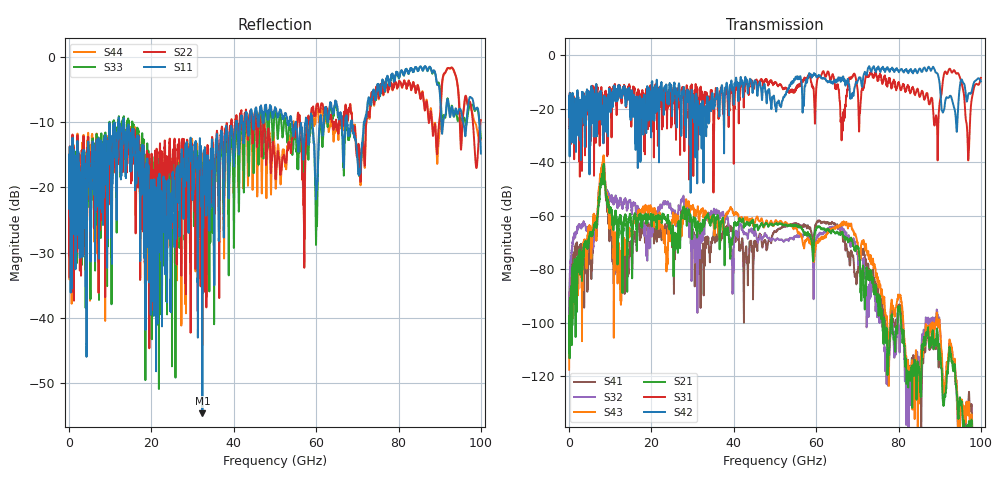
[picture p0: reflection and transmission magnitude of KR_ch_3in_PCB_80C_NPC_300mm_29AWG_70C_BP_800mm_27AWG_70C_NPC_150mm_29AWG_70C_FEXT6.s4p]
# Hz S RI R 45
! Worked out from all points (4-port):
!   4000 points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, 25 MHz to 100 GHz, reference 45 ohm
!   strongest paths, dB at 25 MHz, 25.02 GHz, 50.02 GHz, 75.03 GHz, 100 GHz:
!     S42: -20.7, -20.7, -18.8, -4.2, -9.7
!     S31: -20.7, -20.9, -10.3, -8.7, -8.4
!     S21: -108.7, -69.4, -63.1, -91.8, -168.8
!     S43: -117.6, -62.4, -62.1, -83.6, -162.1
!     S32: -98.5, -59.0, -69.4, -93.4, -184.6
!     S41: -105.2, -70.2, -66.1, -87.1, -162.5
!   lowest |S11| = -54.6 dB at 32.38 GHz (marker M1), VSWR 1.00, Z = 45.2 - j0.00783 ohm
!   |S11| at or under -10 dB: start of sweep to 12.06 GHz; 13.32 GHz to 40.53 GHz (27.21 GHz wide, 101 % of centre); 68.67 GHz to 71.58 GHz (2.909 GHz wide, 4.15 % of centre)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
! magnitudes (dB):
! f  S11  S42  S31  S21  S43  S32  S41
! 25 MHz  -16.6  -20.7  -20.7  -108.7  -117.6  -98.5  -105.2
! 8.1 GHz  -15.8  -19.0  -16.3  -47.6  -42.6  -45.8  -44.3
! 12.38 GHz  -11.9  -15.0  -12.8  -59.7  -80.2  -53.4  -81.7
! 32.38 GHz  -54.6  -18.2  -21.5  -64.4  -57.9  -68.7  -75.0
! 92.53 GHz  -9.2  -15.1  -5.0  -110.2  -107.0  -108.9  -108.0
! 96.88 GHz  -7.6  -15.0  -37.6  -139.0  -134.3  -143.9  -130.3
! 100 GHz  -14.8  -9.7  -8.4  -168.8  -162.1  -184.6  -162.5
